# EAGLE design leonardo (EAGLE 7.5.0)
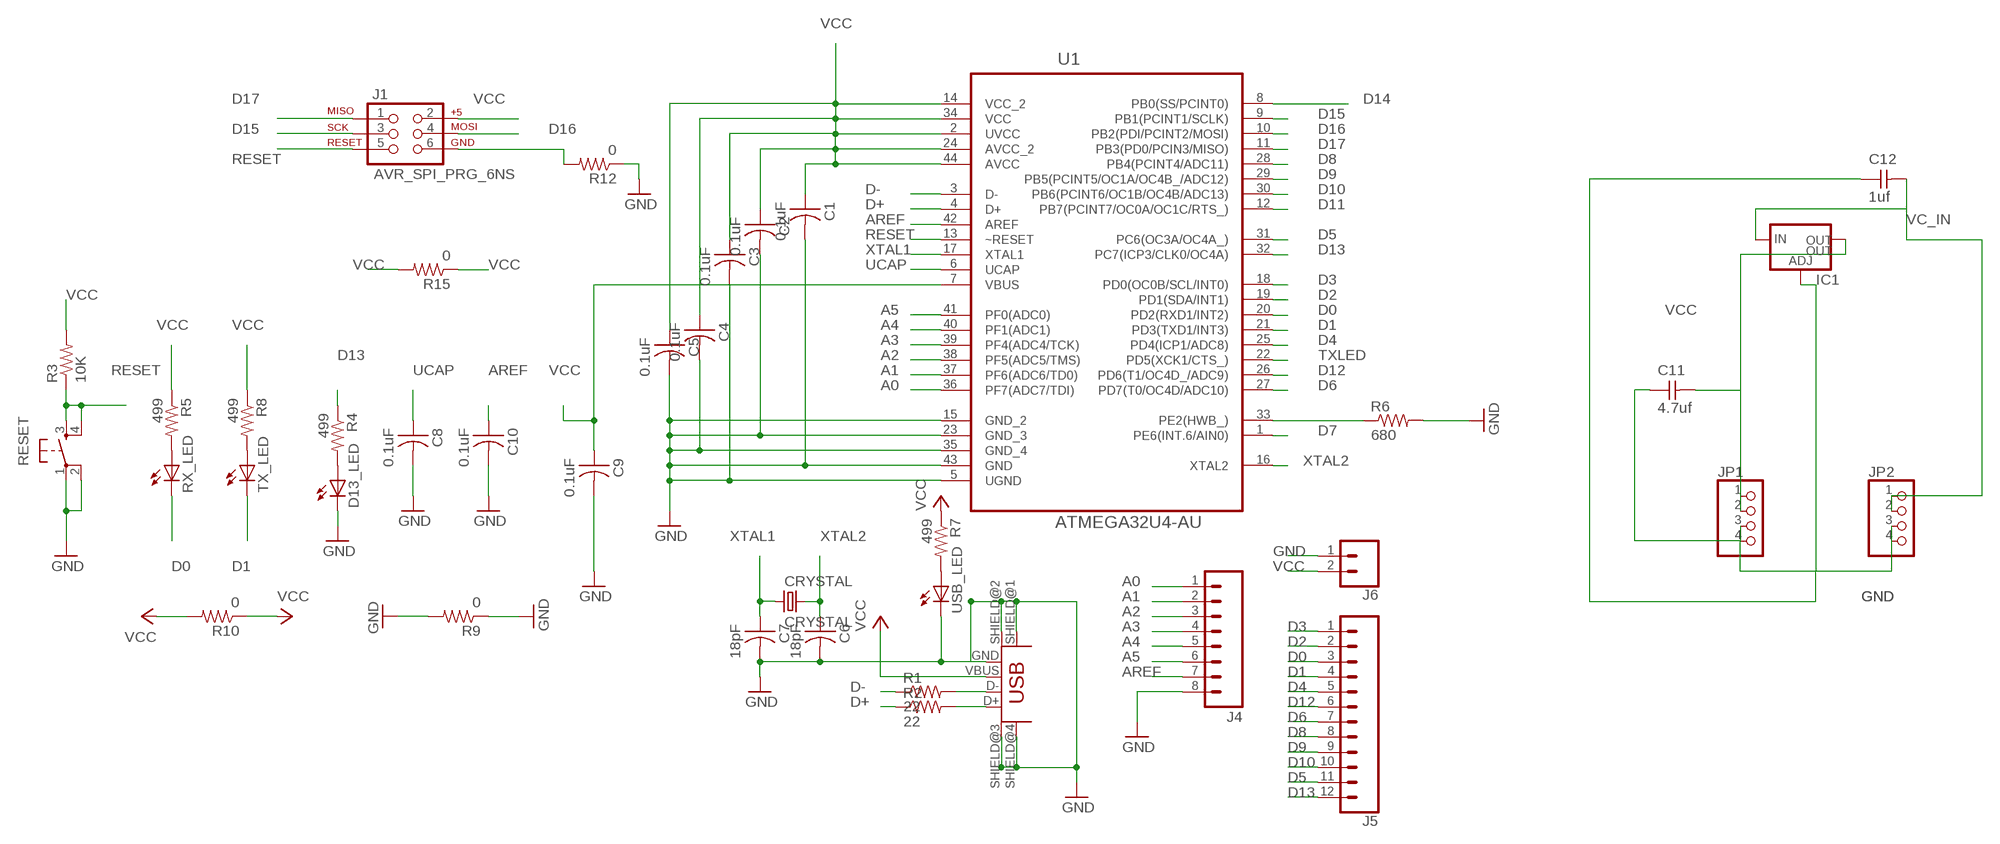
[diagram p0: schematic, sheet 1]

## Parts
C1  0.1uF  CAP-US1206FAB  [C1206FAB]
C2  0.1uF  CAP-US1206FAB  [C1206FAB]
C3  0.1uF  CAP-US1206FAB  [C1206FAB]
C4  0.1uF  CAP-US1206FAB  [C1206FAB]
C5  0.1uF  CAP-US1206FAB  [C1206FAB]
C6  18pF  CAP-US1206FAB  [C1206FAB]
C7  18pF  CAP-US1206FAB  [C1206FAB]
C8  0.1uF  CAP-US1206FAB  [C1206FAB]
C9  0.1uF  CAP-US1206FAB  [C1206FAB]
C10  0.1uF  CAP-US1206FAB  [C1206FAB]
C11  4.7uf  CAP-UNPOLARIZEDFAB  [C1206FAB]
C12  1uf  CAP-UNPOLARIZEDFAB  [C1206FAB]
CRYSTAL  CRYSTAL  [2-SMD-5X3MM]
D13_LED  LED1206  [1206]
IC1  V_REG_LM1117SOT223  [SOT223]
J1  AVR_SPI_PRG_6NS  [2X3-NS]
J4  M08NO_SILK  [1X08_PIN1_NO_SILK]
J5  CONN_12NO_SILK  [1X12_NO_SILK]
J6  CONN_021X02_NO_SILK  [1X02_NO_SILK]
JP1  PINHD-1X4  [1X04]
JP2  PINHD-1X4  [1X04]
R1  22  RES-US1206FAB  [R1206FAB]
R2  22  RES-US1206FAB  [R1206FAB]
R3  10K  RES-US1206FAB  [R1206FAB]
R4  499  RESISTOR1206  [1206]
R5  499  RESISTOR1206  [1206]
R6  680  RES-US1206FAB  [R1206FAB]
R7  499  RESISTOR1206  [1206]
R8  499  RESISTOR1206  [1206]
R9  0  RES-US1206FAB  [R1206FAB]
R10  0  RES-US1206FAB  [R1206FAB]
R12  0  RES-US1206FAB  [R1206FAB]
R15  0  RES-US1206FAB  [R1206FAB]
RESET  6MM_SWITCH6MM_SWITCH  [6MM_SWITCH]
RX_LED  LED1206  [1206]
TX_LED  LED1206  [1206]
U1  ATMEGA32U4-AU  [QFP80P1200X1200X120-44N]
USB_LED  LED1206  [1206]
USB_UPLOAD  USB_MINIB  [USB_MINIB]

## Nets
A0: J4.1 U1.36(PF7(ADC7/TDI))
A1: J4.2 U1.37(PF6(ADC6/TD0))
A2: J4.3 U1.38(PF5(ADC5/TMS))
A3: J4.4 U1.39(PF4(ADC4/TCK))
A4: J4.5 U1.40(PF1(ADC1))
A5: J4.6 U1.41(PF0(ADC0))
AREF: C10.1 J4.7 U1.42(AREF)
D0: J5.3 RX_LED.2(C) U1.20(PD2(RXD1/INT2))
D1: J5.4 TX_LED.2(C) U1.21(PD3(TXD1/INT3))
D2: J5.2 U1.19(PD1(SDA/INT1))
D3: J5.1 U1.18(PD0(OC0B/SCL/INT0))
D4: J5.5 U1.25(PD4(ICP1/ADC8))
D5: J5.11 U1.31(PC6(OC3A/OC4A_))
D6: J5.7 U1.27(PD7(T0/OC4D/ADC10))
D7: U1.1(PE6(INT.6/AIN0))
D8: J5.8 U1.28(PB4(PCINT4/ADC11))
D9: J5.9 U1.29(PB5(PCINT5/OC1A/OC4B_/ADC12))
D10: J5.10 U1.30(PB6(PCINT6/OC1B/OC4B/ADC13))
D11: U1.12(PB7(PCINT7/OC0A/OC1C/RTS_))
D12: J5.6 U1.26(PD6(T1/OC4D_/ADC9))
D13: J5.12 R4.1 U1.32(PC7(ICP3/CLK0/OC4A))
D14: U1.8(PB0(SS/PCINT0))
D15: J1.3 U1.9(PB1(PCINT1/SCLK))
D16: J1.4 U1.10(PB2(PDI/PCINT2/MOSI))
D17: J1.1 U1.11(PB3(PD0/PCIN3/MISO))
D+: R2.1 U1.4(D+)
D-: R1.1 U1.3(D-)
GND: C1.2 C2.2 C3.2 C4.2 C5.2 C6.2 C7.2 C8.2 C9.2 C10.2 C11.1 C12.1 D13_LED.2(C) IC1.1(ADJ) J4.8 J6.1 JP1.3 JP1.4 JP2.3 JP2.4 R6.2 R9.1 R9.2 R12.1 RESET.1(P) RESET.2(P1) U1.5(UGND) U1.15(GND_2) U1.23(GND_3) U1.35(GND_4) U1.43(GND) USB_LED.2(C) USB_UPLOAD.GND USB_UPLOAD.SHIELD@1(SHIELD) USB_UPLOAD.SHIELD@2(SHIELD1) USB_UPLOAD.SHIELD@3(SHIELD2) USB_UPLOAD.SHIELD@4(SHIELD3)
N$1: R1.2 USB_UPLOAD.D-
N$2: R2.2 USB_UPLOAD.D+
N$3: D13_LED.1(A) R4.2
N$4: R5.2 RX_LED.1(A)
N$5: R7.2 USB_LED.1(A)
N$6: R8.2 TX_LED.1(A)
N$13: J1.6 R12.2
N$35: R6.1 U1.33(PE2(HWB_))
RESET: J1.5 R3.1 RESET.3(S) RESET.4(S1) U1.13(~RESET)
TXLED: U1.22(PD5(XCK1/CTS_))
UCAP: C8.1 U1.6(UCAP)
VC_IN: C12.2 IC1.3(IN) JP2.1 JP2.2
VCC: C1.1 C2.1 C3.1 C4.1 C5.1 C9.1 C11.2 IC1.2(OUT) IC1.4(OUT) J1.2 J6.2 JP1.1 JP1.2 R3.2 R5.1 R7.1 R8.1 R10.1 R10.2 R15.1 R15.2 U1.2(UVCC) U1.7(VBUS) U1.14(VCC_2) U1.24(AVCC_2) U1.34(VCC) U1.44(AVCC) USB_UPLOAD.VBUS
XTAL1: C7.1 CRYSTAL.P$1 U1.17(XTAL1)
XTAL2: C6.1 CRYSTAL.P$2 U1.16(XTAL2)

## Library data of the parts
C1-C10 = fab:CAP-US
C11 C12 = fab:CAP-UNPOLARIZED
CRYSTAL = fab:CRYSTAL
D13_LED RX_LED TX_LED USB_LED = ng:LED
IC1 = fab:V_REG_LM1117: Voltage Regulator LM1117 Standard adjustable voltage regulator but in SMD form. Spark Fun Electronics SKU : COM-00595; PROD_ID: VREG-08170
J1 = SparkFun-ConnectorsModified:AVR_SPI_PRG_6: AVR ISP 6 Pin This is the reduced ISP connector for AVR programming. Common on Arduino. This footprint will take up less PCB space and can be used with a 10-pin to 6-pin adapter such as SKU: BOB-08508 **Special note about "TEST_POINT" package. The stop mask is on the top side, so if you want your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
J4 = SparkFun-ConnectorsModified:M08: Header 8 Standard 8-pin 0.1" header. Use with straight break away headers (SKU : PRT-00116), right angle break away headers (PRT-00553), swiss pins (PRT-00743), machine pins (PRT-00117), and female headers (PRT-00115).
J5 = SparkFun-Connectors:CONN_12: Multi connection point. Often used as Generic Header-pin footprint for 0.1 inch spaced/style header connections On any of the 0.1 inch spaced packages, you can populate with these: Break Away Headers - Straight (PRT-00116) Break Away Male Headers - Right Angle (PRT-00553) Female Headers (PRT-00115)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
J6 = SparkFun-Connectors:CONN_02: Multi connection point. Often used as Generic Header-pin footprint for 0.1 inch spaced/style header connections
JP1 JP2 = pinhead:PINHD-1X4: PIN HEADER
R1-R3 R6 R9 R10 R12 R15 = fab:RES-US: Resistor (US Symbol)
R4 R5 R7 R8 = ng:RESISTOR
RESET = fab:6MM_SWITCH: OMRON SWITCH
U1 = Atmel_By_element14_Batch_1:ATMEGA32U4-AU: 8-bit Microcontroller with ISP Flash and USB Controller; MPN: ATMEGA32U4-AU; OC_FARNELL: 1748525; OC_NEWARK: 26R5633; PACKAGE: TQFP-44; SUPPLIER: Atmel
USB_UPLOAD = fab:USB_MINIB

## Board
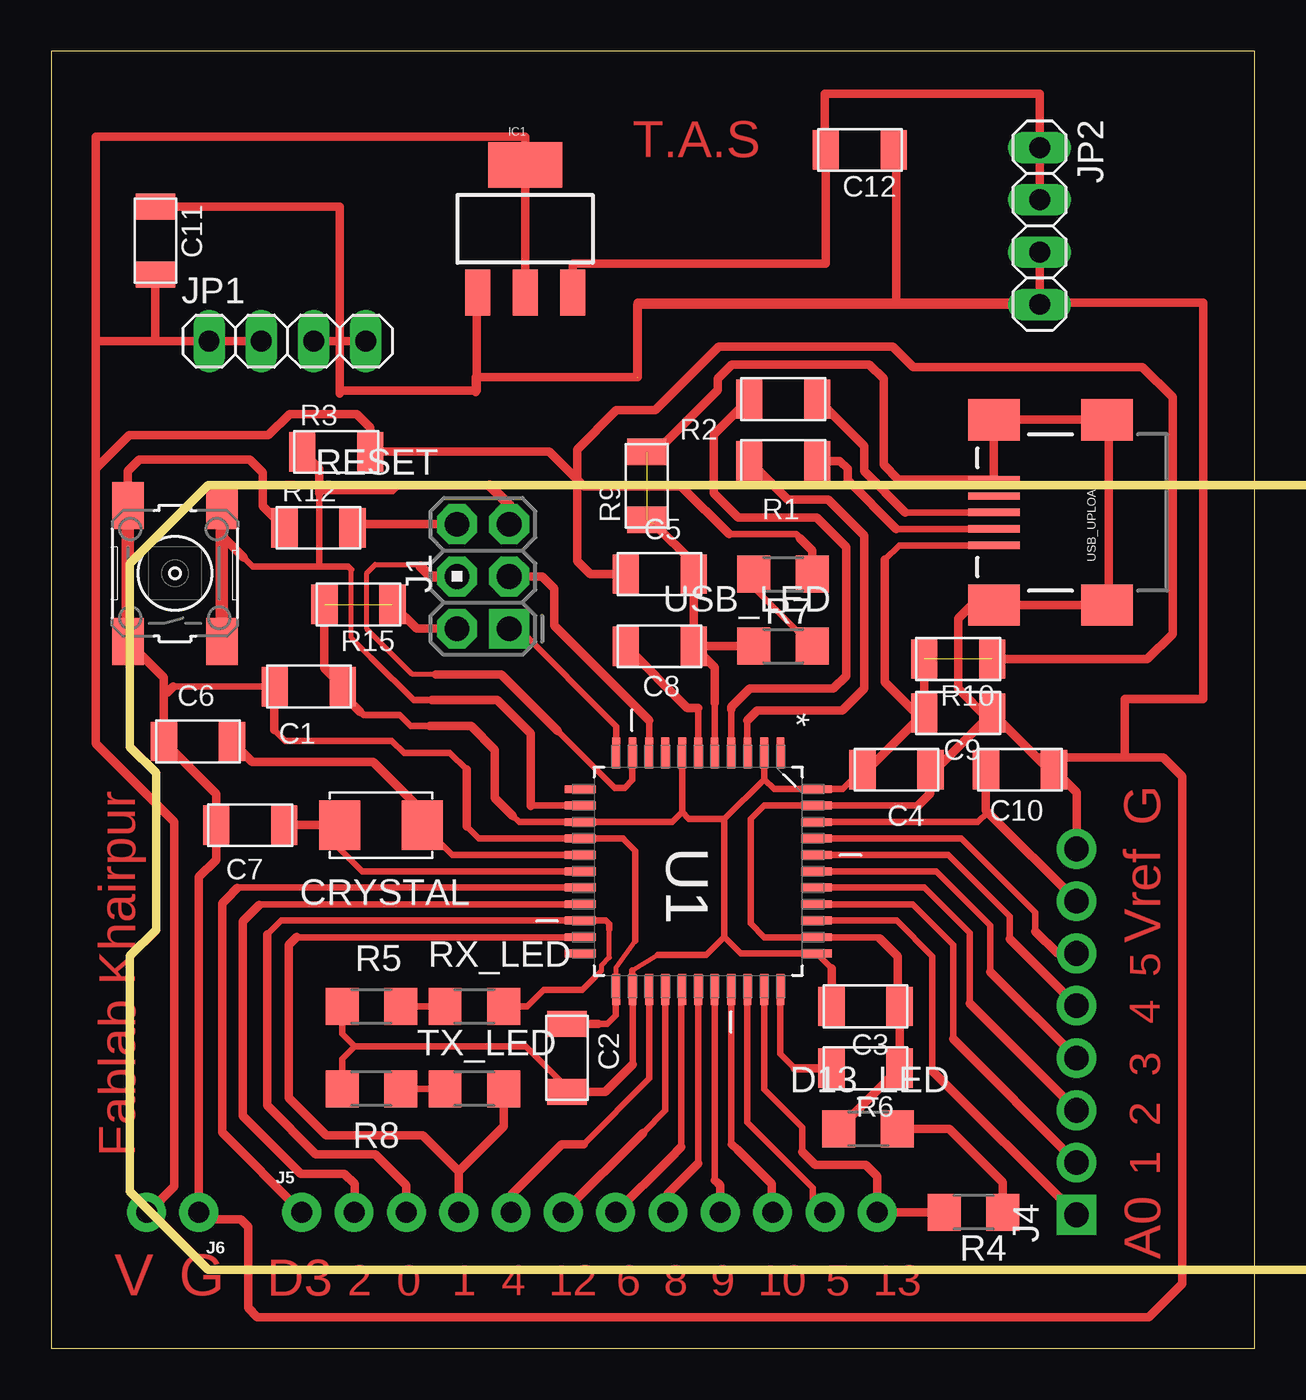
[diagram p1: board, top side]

Size 58.42 x 62.98 mm. Coordinates in mm from the lower left corner, seen from the top.
Outline: 0,0 58.42,0 58.42,62.98 0,62.98 0,0
Copper layers (1*16): Top 0.035mm / dielectric 1.5mm / Bottom 0.035mm
Design rules "default *": minimum track width 10mil, minimum drill 24mil, track to track 0.4mm, track to pad 0.4mm, pad to pad 0.4mm, via to via 0.4mm, smd to smd 0.4mm, copper to edge 40mil, drill to drill 0.4mm, minimum pad ring 10mil, minimum via ring 8mil, stop-mask expansion 4mil, vias tented up to drill 0mil, thermal gap 10mil
Milling: area 3.8,3.8 to 104.1,41.9

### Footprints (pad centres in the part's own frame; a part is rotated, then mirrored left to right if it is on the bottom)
C1206FAB = smd 1.27 x 1.905: 1 -1.651,0; 2 1.651,0
2-SMD-5X3MM = smd 2 x 2.4: P$1 -2,0; P$2 2,0
1206 = smd 1.6 x 1.803: 1 -1.422,0; 2 1.422,0
SOT223 = smd 1.219 x 2.235: 1 -2.311,-3.099; 2 0,-3.099; 3 2.311,-3.099 | smd 3.6 x 2.2: 4 0,3.099
2X3-NS = drill 1.2 pad 1.93 square: 1 -2.54,-1.27 | drill 1.2 pad 1.93 octagon: 2 -2.54,1.27; 3 0,-1.27; 4 0,1.27; 5 2.54,-1.27; 6 2.54,1.27
1X08_PIN1_NO_SILK = drill 1.2 pad 1.93 square: 1 0,0 | drill 1.2 pad 1.93: 2 2.54,0; 3 5.08,0; 4 7.62,0; 5 10.16,0; 6 12.7,0; 7 15.24,0; 8 17.78,0
1X12_NO_SILK = drill 1.016 pad 1.88: 1 0,0; 2 2.54,0; 3 5.08,0; 4 7.62,0; 5 10.16,0; 6 12.7,0; 7 15.24,0; 8 17.78,0; 9 20.32,0; 10 22.86,0; 11 25.4,0; 12 27.94,0
1X02_NO_SILK = drill 1.016 pad 1.88: 1 0,0; 2 2.54,0
1X04 = drill 1.016 long: 1 -3.81,0; 2 -1.27,0; 3 1.27,0; 4 3.81,0
R1206FAB = smd 1.27 x 1.905: 1 -1.651,0; 2 1.651,0
6MM_SWITCH = smd 2.286 x 1.524: 1 -3.302,2.286; 2 3.302,2.286; 3 -3.302,-2.286; 4 3.302,-2.286
QFP80P1200X1200X120-44N = smd 1.5 x 0.38: 1 -5.74,3.988; 2 -5.74,3.2; 3 -5.74,2.388; 4 -5.74,1.6; 5 -5.74,0.787; 6 -5.74,0; 7 -5.74,-0.787; 8 -5.74,-1.6; 9 -5.74,-2.388; 10 -5.74,-3.2; 11 -5.74,-3.988; 23 5.74,-3.988; 24 5.74,-3.2; 25 5.74,-2.388; 26 5.74,-1.6; 27 5.74,-0.787; 28 5.74,0; 29 5.74,0.787; 30 5.74,1.6; 31 5.74,2.388; 32 5.74,3.2; 33 5.74,3.988 | smd 0.38 x 1.5: 12 -3.988,-5.74; 13 -3.2,-5.74; 14 -2.388,-5.74; 15 -1.6,-5.74; 16 -0.787,-5.74; 17 0,-5.74; 18 0.787,-5.74; 19 1.6,-5.74; 20 2.388,-5.74; 21 3.2,-5.74; 22 3.988,-5.74; 34 3.988,5.74; 35 3.2,5.74; 36 2.388,5.74; 37 1.6,5.74; 38 0.787,5.74; 39 0,5.74; 40 -0.787,5.74; 41 -1.6,5.74; 42 -2.388,5.74; 43 -3.2,5.74; 44 -3.988,5.74
USB_MINIB = smd 2.5 x 0.35: D+ 3.77,0; D- 3.77,0.8; GND 3.77,-1.6; ID 3.77,-0.8; VBUS 3.77,1.6 | smd 2.5 x 2: SHIELD@1 -1.73,-4.5; SHIELD@2 -1.73,4.5; SHIELD@3 3.77,4.5; SHIELD@4 3.77,-4.5

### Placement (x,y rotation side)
C1  12.5,32.13 180 top
C2  25.03,14.09 90 top
C3  39.53,16.59 0 top
C4  41.03,28.09 0 top
C5  29.53,37.59 0 top
C6  7.11,29.46 180 top
C7  9.65,25.4 180 top
C8  29.53,34.09 0 top
C9  44.03,30.84 0 top
C10  47.03,28.09 0 top
C11  5.05,53.8 270 top
C12  39.25,58.2 180 top
CRYSTAL  16,25.4 0 top
D13_LED  39.66,10.66 180 top
IC1  23,54.37 0 top
J1  20.96,37.48 90 top
J4  49.78,6.47 90 top
J5  12.16,6.59 0 top
J6  7.16,6.59 180 top
JP1  11.46,48.92 0 top
JP2  47.99,54.51 270 top
R1  35.53,43.09 0 top
R2  35.53,46.09 0 top
R3  13.83,43.54 0 top
R4  44.78,6.59 0 top
R5  15.53,16.59 0 top
R6  39.53,13.59 0 top
R7  35.53,37.59 180 top
R8  15.53,12.59 0 top
R9  28.9,41.88 90 top
R10  44.03,33.47 180 top
R12  12.97,39.84 0 top
R15  14.91,36.12 180 top
RESET  5.99,37.63 90 top
RX_LED  20.53,16.59 0 top
TX_LED  20.53,12.59 0 top
U1  31.41,23.16 270 top
USB_LED  35.53,34.09 180 top
USB_UPLOAD  49.53,40.59 180 top

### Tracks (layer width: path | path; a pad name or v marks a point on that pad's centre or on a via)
A0
  Top 0.305: U1.36 41.04,20.77 42.78,19.03 42.78,13.47
  Top 0.406: 42.78,13.47 J4.1
A1
  Top 0.305: U1.37 41.82,21.56 43.78,19.59 43.78,15.01
  Top 0.406: 43.78,15.01 J4.2
A2
  Top 0.305: U1.38 42.38,22.37 44.59,20.16 44.59,16.74
  Top 0.406: 44.59,16.74 J4.3
A3
  Top 0.305: U1.39 42.97,23.16 45.59,20.53 45.59,18.28
  Top 0.406: 45.59,18.28 J4.4
A4
  Top 0.305: U1.40 43.55,23.95 46.53,20.97 46.53,19.88
  Top 0.406: 46.53,19.88 J4.5
A5
  Top 0.305: U1.41 44.19,24.76 47.78,21.17 47.78,20.25
  Top 0.406: 47.78,20.25 48.86,19.17 J4.6
AREF
  Top 0.305: U1.42 44.98,25.55 45.46,26.03
  Top 0.406: J4.7 45.46,26.03 45.38,26.11 C10.1
D0
  Top 0.254: 26.39,18.02 26.72,18.34 26.72,18.59 27.09,18.97 27.09,20.34
  Top 0.305: 10.47,20.09 11.16,20.78 U1.20 25.68,20.78 26.91,20.78 27.09,20.59 27.09,20.34 | RX_LED.2 23.09,16.59 23.91,17.41 25.78,17.41 26.39,18.02
  Top 0.406: 10.47,20.09 10.47,11.78 12.84,9.41 15.72,9.41 17.22,7.91 17.22,6.61 J5.3 17.28,6.59
D1
  Top 0.305: 11.91,19.97 11.92,19.96 U1.21
  Top 0.406: 11.91,19.97 11.53,19.59 11.53,12.16 13.34,10.34 18.03,10.34 19.78,8.59 | 19.78,8.59 J5.4 | TX_LED.2 21.95,10.77 19.78,8.59
D2
  Top 0.305: U1.19 10.12,21.56 9.75,21.19
  Top 0.406: 10.09,21.53 9.75,21.19 9.28,20.72 9.28,11.28 12.09,8.47 14.22,8.47 14.72,7.97 14.72,6.62 J5.2
D3
  Top 0.305: 8.52,21.83 9.06,22.37 U1.18
  Top 0.406: 9.03,22.34 8.52,21.83 8.28,21.59 8.28,10.47 J5.1
D4
  Top 0.305: U1.25 29.03,13.09 25.84,9.91
  Top 0.406: J5.5 22.32,7.44 24.78,9.91 25.84,9.91
D5
  Top 0.305: U1.31 33.78,17.4 33.78,10.97 36.97,7.78 36.97,7.18 J5.11
D6
  Top 0.305: U1.27 30.59,17.39 30.59,9.78
  Top 0.406: J5.7 30.02,9.2 30.59,9.78
D8
  Top 0.305: 31.41,8.97 U1.28
  Top 0.406: 31.41,8.97 29.91,7.47 29.91,6.62 J5.8
D9
  Top 0.305: U1.29 32.22,17.4 32.22,8.16
  Top 0.406: J5.9 32.48,7.9 32.36,8.02 32.22,8.16
D10
  Top 0.305: 33.3,9.64 33.01,9.93 U1.30
  Top 0.406: 33.03,9.91 33.3,9.64 34.97,7.97 34.97,6.64 J5.10
D12
  Top 0.305: U1.26 29.81,11.55 28.73,10.46
  Top 0.406: J5.6 28.73,10.46
D13
  Top 0.305: 36.47,9.53 36.47,10.72 34.61,12.58 U1.32
  Top 0.406: R4.1 J5.12 40.09,8.34 39.53,8.91 37.09,8.91 36.47,9.53
D15
  Top 0.305: U1.9 29.02,30.48
  Top 0.406: J1.3 23.83,37.48 24.41,36.91 24.41,35.09 29.02,30.48
D16
  Top 0.254: 18.66,32.72 17.53,32.72 15.31,34.94 15.31,37.66 15.72,38.06 17.84,38.06 17.94,37.97 18.06,37.84
  Top 0.305: U1.10 28.21,27.59 27.84,27.22 27.34,27.22 24.59,29.97
  Top 0.406: 24.59,29.97 21.84,32.72 18.66,32.72
  Top 0.508: J1.4 18.43,37.48 17.94,37.97
D17
  Top 0.305: U1.11 27.42,30.2 22.68,34.94 J1.1
D+
  Top 0.305: U1.4 33.01,31.01
  Top 0.406: 33.01,31.01 33.01,31.14 33.91,32.03 37.97,32.03 38.59,32.66 38.59,38.91 37.16,40.34 33.34,40.34 32.16,41.53 32.16,44.37 R2.1
D-
  Top 0.305: U1.3 33.8,30.49
  Top 0.406: R1.1 35.76,41.22 37.72,41.22 39.47,39.47 39.47,32.03 38.41,30.97 34.28,30.97 33.8,30.49
GND  (3 unrouted)
  Top 0.254: U1.23 27.42,18.49 28.34,19.78
  Top 0.305: U1.5 32.2,31.32 32.22,31.34 | 20.16,25.34 20.74,24.76 U1.15 27.76,24.76 27.76,24.74 28.34,24.16 28.34,19.78 | RESET.1 4.22,33.82 | 42.09,26.36 U1.43 34.61,26.36 33.95,25.7 33.95,20.62 34.61,19.96 U1.35 40.17,19.96 40.22,19.91 | 26.56,15.74 27,15.74 27.41,16.16 27.41,17.4 U1.23 | C1.2 5.91,32.13 | 20.16,28.09 19.34,28.91 17.12,28.91 16.53,29.5 11.34,29.5 10.81,30.03
  Top 0.406: 40.22,19.91 41.09,19.03 41.09,16.68 C3.2 R6.2 D13_LED.2 | 51.09,36.09 USB_UPLOAD.SHIELD@3 44.69,36.09 44.03,35.44 44.03,32.03 45.45,30.61 | 51.09,36.09 USB_UPLOAD.SHIELD@2 | RESET.2 3.71,42.59 4.27,43.16 9.62,43.16 10.25,42.53 10.25,40.91 R12.1 | C2.2 26.56,15.74 | 32.22,31.34 32.22,33.06 C8.2 | C8.2 USB_LED.2 | C8.2 C5.2 31.18,38.13 29.28,40.03 | 20.16,25.34 20.16,28.09 | J4.8 49.78,27 C10.2 48.43,28.09 47.85,28.68 | 47.85,28.68 C9.2 45.45,30.61 | 45.45,30.61 42.93,28.09 C4.2 42.68,26.95 42.09,26.36 | 7.22,6.53 J6.1 | 51.09,36.09 51.34,36.34 51.34,45.01 USB_UPLOAD.SHIELD@1 USB_UPLOAD.SHIELD@4 USB_UPLOAD.GND 41.12,42.19 40.41,42.91 40.41,47.09 39.72,47.78 33.03,47.78 32.34,47.09 32.34,46.53 29.35,43.53 R9.2 | 10.81,30.03 10.81,32.09 C1.2 | J6.1 7.5,6.25 9.19,6.25 9.55,5.89 9.55,1.95 10,1.5 53.28,1.5 54.91,3.12 54.91,27.77 54,28.68 52.12,28.68 | 52.12,28.68 47.85,28.68 | 5.46,31.81 C6.2 8,26.92 C7.2 8,23.72 7.16,22.88 J6.1 | 5.46,31.81 5.46,32.58 4.22,33.82 | 5.91,32.13 5.6,31.81 5.46,31.81 | JP1.4 14,48.92 | JP2.3 JP2.4 28.44,50.7 28.44,47.16 20.66,47.16 | JP1.3 14,48.92 | 14,48.92 14,46.5 | 14,46.5 14,46.38 | 20.66,47.16 20.66,46.5 14,46.5 | IC1.1 20.66,51.23 20.66,47.16 | 20.59,46.44 20.59,47.16 28.47,47.16 28.47,50.78 41.03,50.78 | 41.03,50.78 55.94,50.78 55.94,31.53 52.12,31.53 52.12,28.68 | C12.1 41.03,58.2 41.03,50.78 | C11.1 14,55.45 14,48.92
  Top 0.61: RESET.1 RESET.2
N$1
  Top 0.305: USB_UPLOAD.D- 41.02,39.79
  Top 0.406: 41.02,39.79 38.66,42.16 38.66,42.72 38.28,43.09 R1.2
N$2
  Top 0.305: USB_UPLOAD.D+ 41.47,40.59
  Top 0.406: 41.47,40.59 39.47,42.59 39.47,43.81 R2.2
N$3
  Top 0.406: R4.2 46.2,8.05 43.59,10.66 D13_LED.1
N$4
  Top 0.305: R5.2 RX_LED.1
N$5
  Top 0.305: R7.2 34.11,36.94 USB_LED.1
N$6
  Top 0.305: R8.2 TX_LED.1
N$13
  Top 0.406: R12.2 14.81,40.03 19.68,40.03
  Top 0.508: 19.68,40.03 J1.6
N$35
  Top 0.305: U1.33 35.4,14.88 35.4,14.48 35.4,14.29 36.09,13.59
  Top 0.406: 36.09,13.59 R6.1
RESET
  Top 0.254: 15.56,33.5 14.56,34.5 14.56,37.81
  Top 0.305: U1.13 23.3,26.36 23.28,26.34 | 18.47,31.47 17.59,31.47 15.56,33.5 | 14.56,37.81 14.41,37.97 13,37.97 | 13,37.97 9.78,37.97 9.34,38.41 | 13,41.5 13,37.97 | 16.84,41.91 16.56,41.62 13.06,41.62 13,41.69
  Top 0.406: RESET.4 8.28,39.47 9.34,38.41 | 23.28,26.34 23.28,29.84 21.66,31.47 18.47,31.47 | 21.28,41.91 16.84,41.91 | R3.1 13,42.72 13,41.69 13,41.5
  Top 0.508: J1.5 22.23,40.96 21.28,41.91
  Top 0.61: RESET.4 RESET.3
UCAP
  Top 0.305: U1.6 31.41,31.09
  Top 0.406: 31.41,31.09 30.88,31.09 C8.1
VC_IN
  Top 0.406: JP2.2 JP2.1 47.99,60.94 37.56,60.94 37.56,58.2 C12.2 37.6,52.69 25.31,52.69 IC1.3
VCC  (2 unrouted)
  Top 0.254: 28.21,18.34 29.44,19.09
  Top 0.305: 32.68,19.97 32.68,25.7 | U1.7 30.62,26.03 | 34.61,27.63 35.09,27.15 U1.44 38.43,27.15 C4.1 | 34.61,27.63 32.68,25.7 | 30.62,26.03 30.14,25.55 U1.14 22.7,25.55 22.41,25.84 | 32.68,25.7 30.96,25.7 30.62,26.03 | 32.68,19.97 33.48,19.17 U1.34 37.88,18.44 | 32.68,19.97 31.81,19.09 29.44,19.09 | 34.61,27.63 U1.2 | 28.22,13.78 U1.24 28.21,18.34 | C2.1 25.03,12.66 23.03,14.66 14.72,14.66 | R5.1 14.11,15.27 14.72,14.66 | R8.1 14.11,14.05 14.72,14.66 | 36.34,39.34 36.16,39.53 32.91,39.53 | USB_UPLOAD.VBUS 41.16,38.99 40.47,38.31 | 15,30.91 15.16,30.75 16.91,30.75 17.44,30.22 18.38,30.22 18.53,30.22
  Top 0.406: C2.1 26.88,12.44 28.22,13.78 | C5.1 26.16,37.59 25.53,38.22 25.53,42.19 | R7.1 36.95,38.73 36.34,39.34 | 32.91,39.53 30.59,41.84 25.88,41.84 25.53,42.19 | C4.1 39.63,28.09 C9.1 | 42.3,30.92 C9.1 | C9.1 42.53,31 42.38,31.15 R10.2 | J6.2 4.72,6.59 5.97,7.84 5.97,25.56 2.16,29.38 2.16,42.72 | 2.16,42.72 3.78,44.34 10.53,44.34 11.56,45.38 14.81,45.38 15.48,44.7 R3.2 24.18,43.54 25.53,42.19 | C9.1 41.97,30.84 40.47,32.34 40.47,38.31 | C3.1 37.88,18.44 | C1.1 | 15,30.91 14.15,31.75 C1.1 | R15.1 17.74,34.94 J1.2 | R15.2 13.26,33.02 C1.1 | 25.53,42.19 25.53,43.66 27.44,45.56 29.31,45.56 32.41,48.66 40.84,48.66 41.84,47.66 52.97,47.66 54.44,46.19 54.44,34.69 53.22,33.47 R10.1 | 22.41,25.84 21.53,26.72 21.53,29.06 20.38,30.22 18.38,30.22 | JP1.1 JP1.2 5.03,48.92 | IC1.4 IC1.2 23,58.84 2.16,58.84 2.16,48.92 | 2.16,48.92 2.16,42.72 | 5.03,48.92 2.16,48.92 | C11.2 5.03,52.14 5.03,48.92
XTAL1
  Top 0.305: U1.17 15.09,23.16 14,24.25 CRYSTAL.P$1
  Top 0.406: C7.1 CRYSTAL.P$1
XTAL2
  Top 0.305: CRYSTAL.P$2 19.46,23.95 U1.16
  Top 0.406: C6.1 9.76,28.47 15.62,28.47 18,26.09 CRYSTAL.P$2

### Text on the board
Top: T.A.S | G | Vref | 5 | 4 | 3 | 2 | Fablab Khairpur | 1 | A0 | V | G | D3 | 2 | 0 | 1 | 4 | 12 | 6 | 8 | 9 | 10 | 5 | 13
